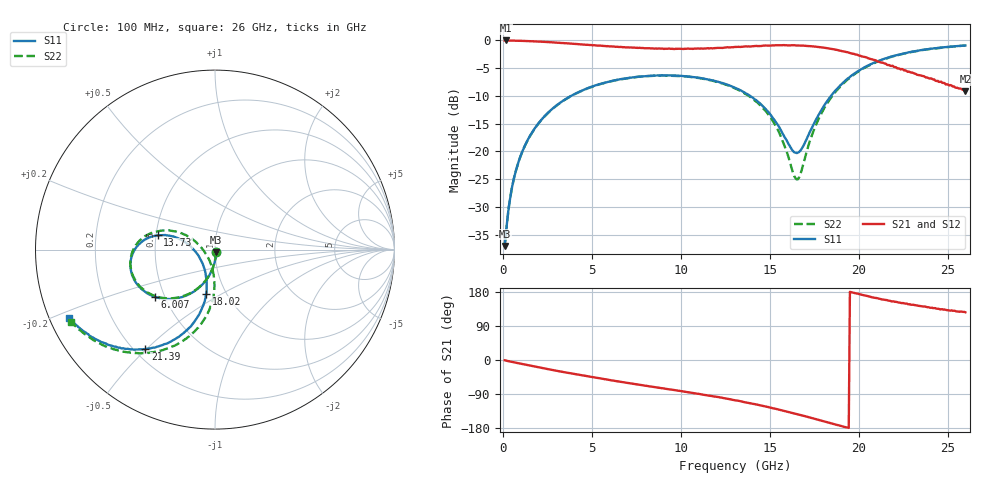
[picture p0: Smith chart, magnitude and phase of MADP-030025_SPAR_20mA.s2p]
!Mean
# HZ S DB R 50
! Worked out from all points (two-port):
!   400 points, 100 MHz to 26 GHz, reference 50 ohm
!   highest |S21| = -0.04 dB at 164.9 MHz (marker M1); lowest = -9.2 dB at 26 GHz (marker M2)
!   |S21| within 3 dB of the highest: start of sweep to 20.38 GHz
!   lowest |S11| = -37.0 dB at 100 MHz (marker M3), VSWR 1.03, Z = 50.5 - j1.32 ohm
!   |S11| at or under -10 dB: start of sweep to 3.841 GHz; 13.9 GHz to 18.45 GHz (4.55 GHz wide, 28.1 % of centre)
!   |S22| runs from -37.0 to -0.9 dB; largest |S21 - S12| = 0.0057
!   S11 on the Smith chart (normalised r, x): 100 MHz: 1.01, -0.03; 6.007 GHz: 0.44, -0.28; 13.73 GHz: 0.51, +0.09; 18.02 GHz: 0.81, -0.43; 21.39 GHz: 0.24, -0.50; 26 GHz: 0.06, -0.22
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1e8  -37.03 -67.9  -0.05 -0.7  -0.05 -0.8  -37.04 -68.7
1.6491e8  -35.09 -73.2  -0.04 -1.5  -0.05 -1.5  -35.08 -73.9
3.5965e8  -29.47 -82.7  -0.06 -3.5  -0.06 -3.5  -29.51 -82.7
6.193e8  -24.89 -88.8  -0.07 -6.1  -0.08 -6.0  -24.93 -89.3
1.3333e9  -18.33 -99.1  -0.13 -12.9  -0.14 -12.9  -18.38 -99.2
2.5667e9  -12.95 -112.2  -0.34 -24.4  -0.34 -24.4  -13.01 -112.5
4.4491e9  -9.04 -129.2  -0.75 -40.6  -0.75 -40.6  -9.07 -129.9
6.007e9  -7.42 -142.0  -1.10 -53.1  -1.10 -53.0  -7.45 -142.8
8.7982e9  -6.33 -162.2  -1.48 -73.4  -1.49 -73.4  -6.37 -163.6
1.1005e10  -6.74 -177.0  -1.48 -89.2  -1.48 -89.3  -6.79 -179.4
1.3082e10  -8.59 169.5  -1.21 -106.5  -1.23 -106.4  -8.70 165.4
1.3732e10  -9.67 166.0  -1.12 -112.3  -1.15 -112.4  -9.84 161.0
1.5289e10  -14.46 164.0  -0.91 -128.2  -0.91 -128.2  -15.14 153.7
1.6523e10  -20.30 -149.9  -0.94 -142.6  -0.94 -142.7  -25.05 -151.0
1.6782e10  -19.61 -131.0  -0.96 -145.8  -0.96 -145.8  -23.54 -118.2
1.7367e10  -15.80 -107.6  -1.08 -153.1  -1.09 -153.0  -17.15 -93.2
1.8016e10  -11.98 -101.2  -1.32 -161.5  -1.33 -161.5  -12.50 -91.1
1.9379e10  -6.90 -107.6  -2.16 -178.5  -2.15 -178.4  -7.06 -102.0
2.1391e10  -3.39 -125.0  -4.08 159.5  -4.07 159.8  -3.45 -121.6
2.1716e10  -3.06 -127.7  -4.45 156.4  -4.45 156.3  -3.11 -124.4
2.3988e10  -1.56 -143.8  -6.90 138.3  -6.83 138.0  -1.58 -141.7
2.6e10  -0.94 -154.9  -9.15 125.9  -9.03 125.9  -0.95 -153.2
